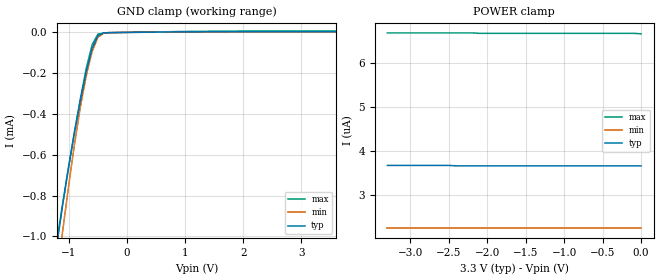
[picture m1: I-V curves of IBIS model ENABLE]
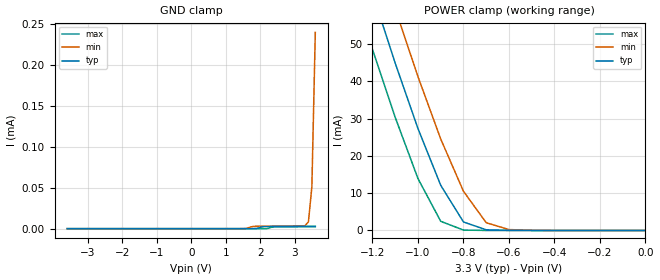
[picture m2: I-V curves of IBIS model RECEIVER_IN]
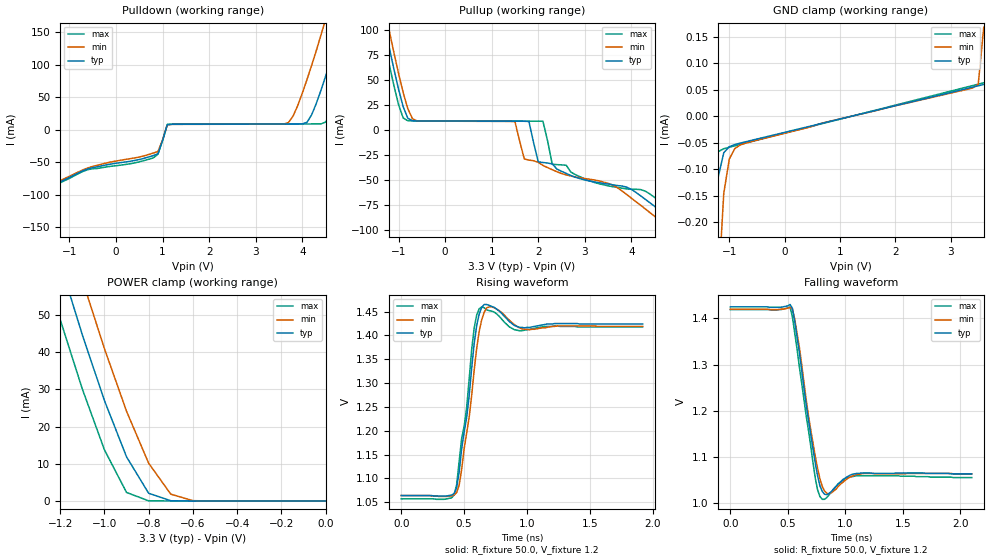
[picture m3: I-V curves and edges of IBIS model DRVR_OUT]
|   Texas Instruments Incorporated
|   Data Transmissions Products
|   IBIS Model for SN65LVDS20
|   8DRF  Small-Outline No-Lead Package
[IBIS Ver]   3.2
[Comment char]   |_char
[File name]   lvds20.ibs
[File Rev]   1.1
[Date]   11Jun04
[Source]   File originated at Texas Instruments Incorporated.
   Data Transmission Products Group.
[Notes]
[Disclaimer]
(C) Copyright Texas Instruments Incorporated 2004
   All rights reserved
  Texas Instruments Incorporated hereby grants the user of this IBIS
model a non-exclusive, nontransferable license to use this IBIS model
under the following terms.  Before using this IBIS model, the user
should read this license.  If the user does not accept these terms,
the IBIS model should be returned to Texas Instruments within 30 days.
  The user is granted this license only to use the IBIS model and
is not granted rights to sell, load, rent, lease or license the IBIS
model in whole or in part, or in modified form to anyone other than
user.  User may modify the IBIS model to suit its specific applications
but rights to derivative works and such modifications shall belong to
Texas Instruments.
  This IBIS model is provided on an "AS IS" basis and Texas Instruments
makes absolutely no warranty with respect to the information contained
herein.  TEXAS INSTRUMENTS DISCLAIMS AND CUSTOMER WAIVES ALL WARRANTIES,
EXPRESS OR IMPLIED, INCLUDING WARRANTIES OF MERCHANTABILITY OR FITNESS
FOR A PARTICULAR PURPOSE. The entire risk as to quality and performance
is with the Customer. ACCORDINGLY, IN NO EVENT SHALL THE COMPANY BE LIABLE
FOR ANY DAMAGES, WHETHER IN CONTRACT OR TORT,INCLUDING ANY LOST PROFITS
OR OTHER INCIDENTAL, CONSEQUENTIAL, EXEMPLARY, OR PUNITIVE DAMAGES ARISING
OUT OF THE USE OR APPLICATION OF THE IBIS model provided in this package.
Further, Texas Instruments reserves the right to discontinue or make changes
without notice to any product herein to improve reliability, function, or
design. Texas Instruments does not convey any license under patent rights
or any other intellectual property rights, including those of third parties.
Contact Texas Instruments at ATTN:DATA TRANSMISSIONS
[Copyright]   Copyright 2004, Texas Instruments, All Rights Reserved
[Component]   LVDS20DRF
[Manufacturer]  Texas Instruments Incorporated
[Package]
|   typ   min   max
R_pkg   0.189   0.176   0.203
L_pkg   0.802nH   0.759nH   0.850nH
C_pkg   0.053pF   0.046pF   0.067pF
[Pin]   signal_name   model_name   R_pin   L_pin   C_pin
1   NC   NC   0.194   0.817n   0.054p
2   A   RECEIVER_IN   0.193   0.814n   0.054p
3   B   RECEIVER_IN   0.187   0.793n   0.052p
4   VBB   POWER   0.194   0.821n   0.054p
5   EN/   ENABLE   0.176   0.759n   0.046p
6   Z   DRVR_OUT   0.188   0.799n   0.051p
7   Y   DRVR_OUT   0.181   0.772n   0.050p
8   VCC   POWER   0.187   0.791n   0.052p
9   GND   GND   0.203   0.850n   0.067p
[Diff_pin]   inv_pin   vdiff   tdelay_typ   tdelay_min   tdelay_max
| The 'A/Y' pin is Diff_pin and the 'B/Z' pin is the inv_pin
2   3   0.100   0 0 0
7   6   0.000   0 0 0
| Models and submodels in the file (3): ENABLE (Input), RECEIVER_IN (Input), DRVR_OUT (3-state)
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|   Enable Input Model
[Model]   ENABLE
Model_type   Input
|Signals   /E
Vinh = 2.0
Vinl = 0.8
C_comp   3.3pF   3.28pF   3.38pF
|   typ   min   max
[Temperature Range]   25   -40   85
[Voltage range]   3.3V   3.0V   3.6V
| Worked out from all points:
|   GND clamp passes 1 mA (typ) near -1.18 V on its own axis
[GND_clamp]
|Voltage I(typ)   I(min)   I(max)
-3.6V     -6.81mA    -7.03mA    -6.59mA
-1.2V     -1.03mA    -1.18mA    -1.01mA
-1.1V     -834uA     -961uA     -829uA
-1V       -652uA     -745uA     -654uA
-900mV    -485uA     -543uA     -484uA
-800mV    -330uA     -362uA     -323uA
-700mV    -191uA     -211uA     -176uA
-600mV    -78.2uA    -93.9uA    -60.7uA
-500mV    -15.7uA    -24.3uA    -8.94uA
-400mV    -2.37uA    -3.64uA    -2.58uA
-300mV    -1.1uA     -901nA     -1.79uA
3.6V      3.66uA     2.24uA     6.67uA
[Power_clamp]
| Note that the[POWER_clamp]voltage table is referenced to Vcc
| and is calculated using Vtable=Vcc - Vmeasured.
|Voltage I(typ)   I(min)   I(max)
-3.3V     3.67uA     2.24uA     6.69uA
-2.5V     3.67uA     2.24uA     6.69uA
-2.4V     3.66uA     2.24uA     6.69uA
-2.2V     3.66uA     2.24uA     6.69uA
-2.1V     3.66uA     2.24uA     6.68uA
-100mV    3.66uA     2.24uA     6.68uA
0V        3.66uA     2.24uA     6.67uA
|   Receiver Input Model
[Model]   RECEIVER_IN
Model_type   Input
|Signals   A, B
Vinh = 2.2
Vinl = 1.8
|   typ   min   max
C_comp   1.0pF   0.98pF   1.10pF
|   typ   min   max
[Temperature Range]   25   -40   85
[Voltage range]   3.3V   3.0V   3.6V
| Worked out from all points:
|   POWER clamp passes 1 mA (typ) near -0.74 V on its own axis
[GND_clamp]
|Voltage I(typ)   I(min)   I(max)
-3.6V     -93.5pA    -92.3pA    -96.3pA
1.5V      -4.04pA    13.2nA     -8.24pA
1.8V      4.55nA     2.8uA      -3.22pA
2.1V      2.52uA     3.01uA     483pA
2.4V      2.64uA     3.1uA      2.1uA
3.3V      2.9uA      3.61uA     2.32uA
3.4V      2.93uA     8.35uA     2.35uA
3.5V      2.96uA     51uA       2.37uA
3.6V      2.99uA     240uA      2.4uA
[Power_clamp]
| Note that the[POWER_clamp]voltage table is referenced to Vcc
| and is calculated using Vtable=Vcc - Vmeasured.
|Voltage   I(typ)   I(min)   I(max)
-3.3V     557mA      575mA      539mA
-1.3V     83.2mA     98.5mA     67.8mA
-1.2V     63.6mA     78.6mA     48.5mA
-1.1V     44.8mA     59.4mA     30.3mA
-1V       27.3mA     41.2mA     13.9mA
-900mV    12.1mA     24.5mA     2.46mA
-800mV    2.28mA     10.5mA     111uA
-700mV    181uA      2.08mA     10.4uA
-600mV    29.5uA     240uA      2.64uA
0V        2.9uA      3.29uA     2.4uA
|   Driver Output Model
[Model]   DRVR_OUT
Model_type   3-state
| Signals   Y, Z
Vmeas = 1.2V   |Reference voltage for timing measurements
Cref = 1pF   |Timing specification test load capacitance value
Rref = 50   |Note: 50 Ohm load; single ended configuration
Vref = 1.20V   |Timing specification test load voltage
|Note: 50 Ohm load; single ended configuration
| variable   typ   min   max
C_comp   1.23pF   1.21pF   1.3pF
|   typ   min   max
[Temperature Range]   25.0   -40.0   85.0
[Voltage range]   3.3V   3.0V   3.6V
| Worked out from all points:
|   slope of the pulldown table from 0 to 0.495 V, typ, clamps not added: 86.5 ohm
|   slope of the pullup table from 0 to 0.495 V, typ, clamps not added: 7.12 kohm
|   GND clamp passes 1 mA (typ) near -1.45 V on its own axis
|   POWER clamp passes 1 mA (typ) near -0.74 V on its own axis
|   rising waveform, R_fixture 50.0, V_fixture 1.2: 20-80 % time 98.3ps typ, 101ps min, 94.2ps max; typ from 1.06 V to 1.42 V
|   falling waveform, R_fixture 50.0, V_fixture 1.2: 20-80 % time 123ps typ, 123ps min, 124ps max; typ from 1.43 V to 1.06 V
[Pulldown]
|Voltage I(typ)   I(min)   I(max)
-3.3V     -161mA     -162mA     -161mA
-700mV    -62.9mA    -61.4mA    -63.9mA
800mV     -39.8mA    -35.9mA    -43.3mA
900mV     -37mA      -33.5mA    -37.6mA
1.1V      7.74mA     7.43mA     8.28mA
3.7V      8.79mA     11mA       8.85mA
4.1V      11.5mA     77.4mA     8.9mA
4.4V      60.9mA     146mA      8.99mA
4.5V      82.6mA     170mA      11.8mA
4.8V      152mA      245mA      65.5mA
5.2V      253mA      349mA      159mA
6.6V      642mA      751mA      537mA
[Pullup]
|Voltage   I(typ)   I(min)   I(max)
| Note that the[Pullup]voltage table is referenced to Vcc
| and is calculated using Vtable=Vcc - Vmeasured.
-3.3V     642mA      661mA      625mA
-1.4V     128mA      146mA      111mA
-1.3V     105mA      122mA      87.8mA
-1V       40.7mA     56.5mA     25.3mA
-800mV    11.5mA     21mA       8.99mA
1.5V      8.51mA     8.03mA     8.63mA
1.8V      8.23mA     -30.4mA    8.59mA
2.1V      -32.8mA    -35.7mA    8.5mA
2.3V      -34.2mA    -40mA      -34.5mA
3.6V      -55.1mA    -55.4mA    -57mA
4.9V      -91.1mA    -102mA     -81.4mA
6.6V      -161mA     -177mA     -146mA
[GND_clamp]
|Voltage   I(typ)   I(min)   I(max)
-3.6V     -79.4mA    -88.2mA    -41.5mA
-1.4V     -676uA     -1.36mA    -215uA
-1.3V     -277uA     -722uA     -90.9uA
-1.2V     -114uA     -328uA     -66.4uA
-1.1V     -68.6uA    -145uA     -61uA
-1V       -57.2uA    -80.4uA    -58.1uA
-900mV    -53.1uA    -60.6uA    -55.5uA
-700mV    -47.8uA    -50.3uA    -50.2uA
700mV     -12.5uA    -12.2uA    -13.2uA
3.4V      55.1uA     53.5uA     58uA
3.5V      57.6uA     60.2uA     60.7uA
3.6V      60.1uA     168uA      63.3uA
[Power_clamp]
| Note that the[POWER_clamp]voltage table is referenced to Vcc
| and is calculated using Vtable=Vcc - Vmeasured.
|Voltage   I(typ)   I(min)   I(max)
-3.3V     622mA      646mA      598mA
-1.3V     84.5mA     100mA      69mA
-1.2V     63.8mA     79.2mA     48.7mA
-1.1V     44.6mA     59.3mA     30.1mA
-1V       27mA       40.9mA     13.8mA
-900mV    11.9mA     24.1mA     2.37mA
-800mV    2.15mA     10.2mA     120uA
-700mV    145uA      1.91mA     82.1uA
-600mV    69.2uA     168uA      79.2uA
0V        52.6uA     43.8uA     63.3uA
[Ramp]
|   typ   min   max
dV/dt_r   0.215/82ps   0.213/100ps   0.217/90ps
dV/dt_f   0.217/100ps   0.214/120ps   0.218/120ps
R_load = 50ohm |Note: The measurement is on a single-ended configuration
|   with 100ohm line-to-line.
[Rising Waveform]
R_fixture = 50.0
V_fixture = 1.2
C_fixture = 0p
L_fixture = 0n
|   V(typ)  V(min)  V(max)
0s        1.064V     1.064V     1.057V
420ps     1.068V     1.065V     1.065V
440ps     1.08V      1.07V      1.086V
460ps     1.112V     1.085V     1.134V
520ps     1.227V     1.195V     1.248V
580ps     1.383V     1.327V     1.416V
640ps     1.459V     1.433V     1.46V
720ps     1.461V     1.46V      1.451V
940ps     1.417V     1.416V     1.41V
1.92ns    1.424V     1.419V     1.418V
[Falling Waveform]
R_fixture = 50.0
V_fixture = 1.2
C_fixture = 0p
L_fixture = 0n
|   V(typ)  V(min)  V(max)
0s        1.425V     1.42V      1.419V
520ps     1.43V      1.424V     1.424V
560ps     1.394V     1.399V     1.369V
680ps     1.18V      1.19V      1.158V
740ps     1.086V     1.101V     1.054V
800ps     1.026V     1.037V     1.009V
860ps     1.022V     1.021V     1.019V
980ps     1.052V     1.046V     1.05V
1.1ns     1.065V     1.063V     1.06V
2.1ns     1.064V     1.064V     1.056V
